|Texas Instruments Incorporated
| Marketing part#   Digital Voltage Range   Package-type   #pins
| DAC60096   3.0-5.5V   BGA   196
[IBIS Ver]   4.1
[File name]   dac60096.ibs
[File Rev]   1.0
[Date]   12/16/2014
[Source]
| Texas Instruments Incorporated.
| 12500 TI Blvd
| Dallas, TX -75243
[Notes]   Revision History:
| Rev 1.0: 12/16/2014
| - Initial version of the model
| - Model generated from simulations in TISPICE
| - C_comp although listed in numerical order of value are
|   obtained from varying PVT conditions. For PVT conditions for
|   each specific value refer the buffer description under
|   respective [Model]. IBIS model user is responsible for using
|   appropriate C_comp to simulate for Signal Integrity.
| - Warnings regarding combined Non-monotonicity of various models have been
|   reviewd and considered minor and can be ignored.
| - Model names with a trailing _3p0 contain the model for
|   3.0V operation. Model names with a trailing _5p5 contain the model
|   for 5.5V operation.
[Disclaimer]
| This model is designed as an aid for customers of Texas Instruments.
| TI and its licensors and suppliers make no warranties, either expressed
| or implied, with respect to this  model, including the warranties of
| merchantability or fitness for a particular purpose. The model is
| provided solely on an "as is" basis. The entire risk as to its quality
| and performance is with the customer.
[Copyright]
 (C) Copyright 2014 Texas Instruments Incorporated.All rights reserved.
|   Device
[Component] DAC60096
[Manufacturer]   TI
[Package]  | 196 BGA
| variable   typ   min   max
R_pkg   0.2   0.16   0.24
L_pkg   1.5nH   1.2nH   1.8nH
C_pkg   0.4pF   0.32pF   0.48pF
[Pin]  signal_name   model_name   R_pin   L_pin   C_pin
A1   DAC13G1   NC   NA   NA   NA
A2   DAC12G1   NC   NA   NA   NA
A3   DAC11G1   NC   NA   NA   NA
A4   DAC10G1   NC   NA   NA   NA
A5   DAC16G2   NC   NA   NA   NA
A6   DAC15G2   NC   NA   NA   NA
A7   DAC14G2   NC   NA   NA   NA
A8   DAC13G3   NC   NA   NA   NA
A9   DAC12G3   NC   NA   NA   NA
A10   DAC11G3   NC   NA   NA   NA
A11   DAC10G3   NC   NA   NA   NA
A12   DAC16G4   NC   NA   NA   NA
A13   DAC15G4   NC   NA   NA   NA
A14   DAC14G4   GND   NA   NA   NA
B1   AVSSG1   NC   NA   NA   NA
B2   DAC9G1   NC   NA   NA   NA
B3   DAC8G1   NC   NA   NA   NA
B4   DAC7G1   NC   NA   NA   NA
B5   ADC17G2   NC   NA   NA   NA
B6   AVSSG2   GND   NA   NA   NA
B7   AVSSG2   GND   NA   NA   NA
B8   AVSSG3   GND   NA   NA   NA
B9   AVSSG3   GND   NA   NA   NA
B10   DAC9G3   NC   NA   NA   NA
B11   DAC8G3   NC   NA   NA   NA
B12   DAC18G4   NC   NA   NA   NA
B13   DAC17G4   NC   NA   NA   NA
B14   AVSSG4   GND   NA   NA   NA
C1   VREFLG1   NC   NA   NA   NA
C2   DAC6G1   NC   NA   NA   NA
C3   DAC18G2   NC   NA   NA   NA
C4   DAC19G2   NC   NA   NA   NA
C5   DAC20G2   NC   NA   NA   NA
C6   VREFLG2   NC   NA   NA   NA
C7   VREFLG2   NC   NA   NA   NA
C8   VREFLG3   NC   NA   NA   NA
C9   VREFLG3   NC   NA   NA   NA
C10   DAC7G3   NC   NA   NA   NA
C11   DAC6G3   NC   NA   NA   NA
C12   DAC19G4   NC   NA   NA   NA
C13   DAC20G4   NC   NA   NA   NA
C14   VREFLG4   NC   NA   NA   NA
D1   VREFHG1   NC   NA   NA   NA
D2   DAC5G1   NC   NA   NA   NA
D3   DAC3G1   NC   NA   NA   NA
D4   DAC323G2   NC   NA   NA   NA
D5   DAC21G2   NC   NA   NA   NA
D6   VREFHG2   NC   NA   NA   NA
D7   VREFHG2   NC   NA   NA   NA
D8   VREFHG3   NC   NA   NA   NA
D9   VREFHG3   NC   NA   NA   NA
D10   AGND   GND   NA   NA   NA
D11   DAC5G3   NC   NA   NA   NA
D12   DAC23G4   NC   NA   NA   NA
D13   DAC21G4   NC   NA   NA   NA
D14   VREFHG4   NC   NA   NA   NA
E1   AVCCG1   POWER   NA   NA   NA
E2   DAC4G1   NC   NA   NA   NA
E3   DAC2G1   NC   NA   NA   NA
E4   DAC1G1   NC   NA   NA   NA
E5   DAC22G2   NC   NA   NA   NA
E6   AVCCG2   POWER   NA   NA   NA
E7   AVCCG2   POWER   NA   NA   NA
E8   AVCCG3   POWER   NA   NA   NA
E9   AVCCG3   POWER   NA   NA   NA
E10   AGND   GND   NA   NA   NA
E11   DAC24G2   NC   NA   NA   NA
E12   DAC4G3   NC   NA   NA   NA
E13   DAC22G4   NC   NA   NA   NA
E14   AVCCG4   POWER   NA   NA   NA
F1   AGND   GND   NA   NA   NA
F2   AGND   GND   NA   NA   NA
F3   STATS   STAT   0.1 1.878nH 0.9pF
F4   RESETB   SDIN   0.025 0.89nH   3.24pF
F5   AGND   GND   NA   NA   NA
F6   AVSSS1   GND   NA   NA   NA
F7   AVCCS1   POWER   NA   NA   NA
F8   AVCCS2   POWER   NA   NA   NA
F9   AVSSS2   GND   NA   NA   NA
F10   AGND   GND   NA   NA   NA
F11   DAC26G2   NC   NA   NA   NA
F12   DAC3G3   NC   NA   NA   NA
F13   DAC24G4   NC   NA   NA   NA
F14   HDAC25G4   NC   NA   NA   NA
G1   REF1   NC   NA   NA   NA
G2   AGND   GND   NA   NA   NA
G3   SDO   SDO   0.025 0.74nH 3.28pF
G4   CSB   SDIN   0.025 0.792nH 4.79pF
G5   AGND   GND   NA   NA   NA
G6   DGND   GND   NA   NA   NA
G7   DVDD   POWER   NA   NA   NA
G8   DVDD   POWER   NA   NA   NA
G9   DGND   GND   NA   NA   NA
G10   AGND   GND   NA   NA   NA
G11   DAC25G2   NC   NA   NA   NA
G12   DAC1G3   NC   NA   NA   NA
G13   DAC2G3   NC   NA   NA   NA
G14   REF2   NC   NA   NA   NA
H1   REFGND1   GND   NA   NA   NA
H2   AGND   GND   NA   NA   NA
H3   SDI   SDIN   0.025 0.790nH   3.11pF
H4   SCLK   SDIN   0.025 1.060nH   3.69pF
H5   CLEARB   SDIN   0.025 0.872nH 3.4pF
H6   DGND   GND   NA   NA   NA
H7   DVDD   POWER   NA   NA   NA
H8   DVDD   POWER   NA   NA   NA
H9   DGND   GND   NA   NA   NA
H10   AGND   GND   NA   NA   NA
H11   DAC26G6   NC   NA   NA   NA
H12   DAC4G5   NC   NA   NA   NA
H13   DAC3G5   NC   NA   NA   NA
H14   REFGND2   NC   NA   NA   NA
J1   AGND   GND   NA   NA   NA
J2   AGND   GND   NA   NA   NA
J3   TRIGG   SDIN   0.025 0.874nH   3.29pF
J4   LDACB   SDIN   0.025 0.911nH   3.26pF
J5   AGND   GND   NA   NA   NA
J6   AVSSS4   GND   NA   NA   NA
J7   AVCCS4   POWER   NA   NA   NA
J8   AVCCS3   POWER   NA   NA   NA
J9   AVSSS3   GND   NA   NA   NA
J10   AGND   GND   NA   NA   NA
J11   DAC25G6   NC   NA   NA   NA
J12   DAC24G6   NC   NA   NA   NA
J13   DAC5G5   NC   NA   NA   NA
J14   HDAC2G5   NC   NA   NA   NA
K1   AVCCG8   POWER   NA   NA   NA
K2   DAC23G8   NC   NA   NA   NA
K3   DAC26G8   NC   NA   NA   NA
K4   DAC2G7   NC   NA   NA   NA
K5   DAC3G7   NC   NA   NA   NA
K6   AVCCG7   POWER   NA   NA   NA
K7   AVCCG7   POWER   NA   NA   NA
K8   AVCCG6   POWER   NA   NA   NA
K9   AVCCG6   POWER   NA   NA   NA
K10   AGND   GND   NA   NA   NA
K11   DAC1G7   NC   NA   NA   NA
K12   DAC23G6   NC   NA   NA   NA
K13   DAC6G5   NC   NA   NA   NA
K14   AVCCG5   POWER   NA   NA   NA
L1   VREFHG8   NC   NA   NA   NA
L2   DAC22G8   NC   NA   NA   NA
L3   DAC24G8   NC   NA   NA   NA
L4   DAC25G8   NC   NA   NA   NA
L5   DAC4G7   NC   NA   NA   NA
L6   VREFHG7   NC   NA   NA   NA
L7   VREFHG7   NC   NA   NA   NA
L8   VREFHG6   NC   NA   NA   NA
L9   VREFHG6   NC   NA   NA   NA
L10   AGND   GND   NA   NA   NA
L11   DAC22G6   NC   NA   NA   NA
L12   DAC21G6   NC   NA   NA   NA
L13   DAC7G5   NC   NA   NA   NA
L14   VREFHG5   NC   NA   NA   NA
M1   VREFLG8   NC   NA   NA   NA
M2   DAC20G8   NC   NA   NA   NA
M3   DAC19G8   NC   NA   NA   NA
M4   DAC21G8   NC   NA   NA   NA
M5   DAC6G7   NC   NA   NA   NA
M6   VREFLG7   NC   NA   NA   NA
M7   VREFLG7   NC   NA   NA   NA
M8   VREFLG6   NC   NA   NA   NA
M9   VREFLG6   NC   NA   NA   NA
M10   DAC5G7   NC   NA   NA   NA
M11   DAC20G6   NC   NA   NA   NA
M12   DAC9G5   NC   NA   NA   NA
M13   DAC8G5   NC   NA   NA   NA
M14   VREFLG5   NC   NA   NA   NA
N1   AVSSG8   GND   NA   NA   NA
N2   DAC18G8   NC   NA   NA   NA
N3   DAC17G8   NC   NA   NA   NA
N4   DAC8G7   NC   NA   NA   NA
N5   DAC9G7   NC   NA   NA   NA
N6   AVSSG7   GND   NA   NA   NA
N7   AVSSG7   GND   NA   NA   NA
N8   AVSSG6   GND   NA   NA   NA
N9   AVSSG6   GND   NA   NA   NA
N10   DAC7G7   NC   NA   NA   NA
N11   DAC18G6   NC   NA   NA   NA
N12   DAC19G6   NC   NA   NA   NA
N13   DAC10G5   NC   NA   NA   NA
N14   AVSSG5   GND   NA   NA   NA
P1   DAC14G8   NC   NA   NA   NA
P2   DAC15G8   NC   NA   NA   NA
P3   DAC16G8   NC   NA   NA   NA
P4   DAC10G7   NC   NA   NA   NA
P5   DAC11G7   NC   NA   NA   NA
P6   DAC12G7   NC   NA   NA   NA
P7   DAC13G7   NC   NA   NA   NA
P8   DAC14G6   NC   NA   NA   NA
P9   DAC15G6   NC   NA   NA   NA
P10   DAC16G6   NC   NA   NA   NA
P11   DAC17G6   NC   NA   NA   NA
P12   DAC11G5   NC   NA   NA   NA
P13   DAC12G5   NC   NA   NA   NA
P14   DAC13G5   NC   NA   NA   NA
|   Model Selectors
[Model Selector]  SDO
SDO_5p5_nom  sdout buffer at 5.5V power, nomal drive strength.
SDO_3p0_nom  sdout buffer at 3.0V power, nomal drive strength.
SDO_5p5_str  sdout buffer at 5.5V power, high drive strength.
SDO_3p0_str  sdout buffer at 3.0V power, high drive strength.
[Model Selector]  SDIN
SDIN_5p5  input buffer at 5.5V power.
SDIN_3p0  input buffer at 3.0V power.
[Model Selector]  STAT
STAT_5p5  STAT buffer at 5.5V power.
STAT_3p0  STAT buffer at 3.0V power.
| Models and submodels in the file (8): SDIN_3p0 (Input), SDIN_5p5 (Input), SDO_3p0_nom (Output), SDO_3p0_str (Output), SDO_5p5_nom (Output), SDO_5p5_str (Output), STAT_3p0 (Output), STAT_5p5 (Output)
